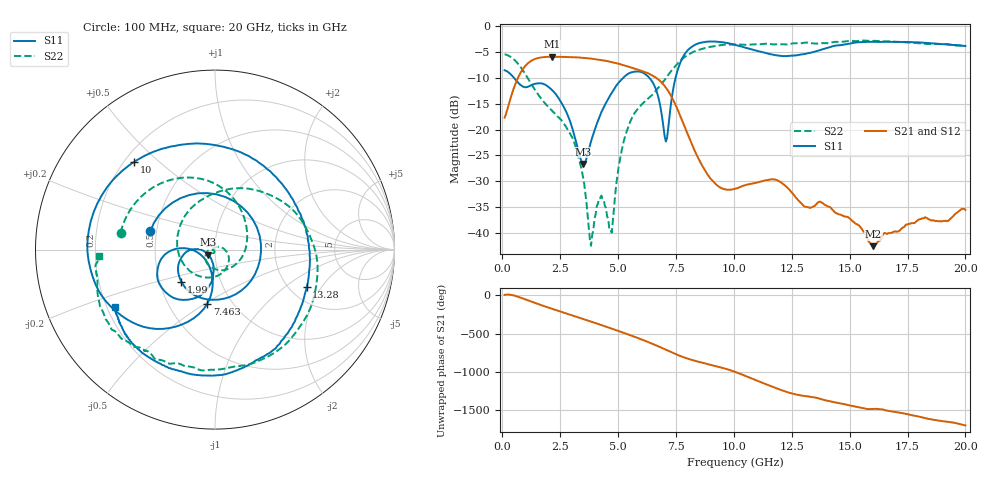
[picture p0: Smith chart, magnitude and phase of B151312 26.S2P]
!  2-Port S-parameters saved by WinCal
! VAR MeasName=S-Parameters (CALIBRATED_DATA) read from VNA (N5244A)
! VAR MeasDate=12/8/2015 5:45:24 PM
! VAR NAME=B151312 26
! VAR FILENAME=B151312 26.S2P
! VAR DATE=12/8/2015 5:45:24 PM
! VAR PHYS_PORTS=1,2
# Hz S DB R 50
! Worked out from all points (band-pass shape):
!   401 points, 100 MHz to 20 GHz, reference 50 ohm
!   highest |S21| = -5.92 dB at 2.14 GHz (marker M1); lowest = -42.6 dB at 16.02 GHz (marker M2)
!   |S21| within 3 dB of the highest: 800.7 MHz to 6.199 GHz (5.398 GHz wide, 154 % of centre)
!   lowest |S11| = -26.7 dB at 3.483 GHz (marker M3), VSWR 1.10, Z = 46.4 - j2.59 ohm
!   |S11| at or under -10 dB: 504.7 MHz to 5.22 GHz (4.715 GHz wide, 165 % of centre); 6.352 GHz to 7.482 GHz (1.13 GHz wide, 16.3 % of centre)
!   |S22| runs from -42.5 to -2.8 dB; largest |S21 - S12| = 0.0015
!   S11 on the Smith chart (normalised r, x): 100 MHz: 0.46, +0.11; 1.99 GHz: 0.65, -0.25; 7.463 GHz: 0.77, -0.51; 10 GHz: 0.24, +0.41; 13.28 GHz: 2.45, -1.48; 20 GHz: 0.23, -0.25
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1e8  -8.52 164.3  -17.71 7.6  -17.71 7.6  -5.43 169.8
9.4575e8  -11.78 7.2  -7.94 -46.2  -7.94 -46.2  -8.92 87.3
1.9905e9  -11.74 -136.3  -5.93 -159.6  -5.92 -159.6  -15.63 -3.4
2.13975e9  -12.31 -147.4  -5.92 -174.6  -5.92 -174.6  -16.28 -19.1
3.43325e9  -26.26 -152.8  -6.10 57.3  -6.09 57.3  -27.85 -171.1
3.483e9  -26.66 -143.1  -6.11 52.4  -6.11 52.3  -29.16 -173.2
3.83125e9  -22.31 -99.2  -6.26 17.2  -6.27 17.2  -42.49 -131.9
4.279e9  -16.63 -94.2  -6.54 -28.7  -6.54 -28.7  -32.76 -121.0
4.677e9  -13.25 -100.7  -6.89 -70.4  -6.87 -70.3  -39.43 136.7
5.672e9  -8.83 -137.3  -8.13 -178.1  -8.13 -178.1  -17.13 -76.0
6.7665e9  -14.25 177.8  -10.40 48.0  -10.41 48.0  -11.76 126.1
7.065e9  -22.31 -142.4  -11.89 6.8  -11.87 6.9  -10.07 91.0
7.463e9  -10.35 -98.0  -15.03 -47.3  -15.03 -47.2  -7.77 53.1
8.70675e9  -3.08 -170.2  -27.55 -168.3  -27.53 -168.4  -4.29 -25.7
1.000025e10  -3.55 132.9  -31.52 83.3  -31.55 82.9  -3.53 -69.3
1.005e10  -3.59 130.8  -31.45 77.7  -31.50 77.2  -3.52 -70.7
1.13435e10  -5.12 70.3  -29.86 -79.5  -29.93 -79.6  -3.40 -95.5
1.328375e10  -5.17 -22.4  -35.18 111.3  -35.09 111.6  -3.22 -119.8
1.338325e10  -5.07 -26.1  -35.01 107.2  -34.97 107.8  -3.30 -121.1
1.602e10  -3.02 -101.8  -42.56 -48.4  -42.45 -47.8  -2.83 -147.5
1.67165e10  -3.03 -113.7  -40.02 -76.1  -39.82 -76.0  -2.91 -153.3
2e10  -3.85 -150.2  -35.54 94.4  -35.60 93.4  -3.75 -176.7
